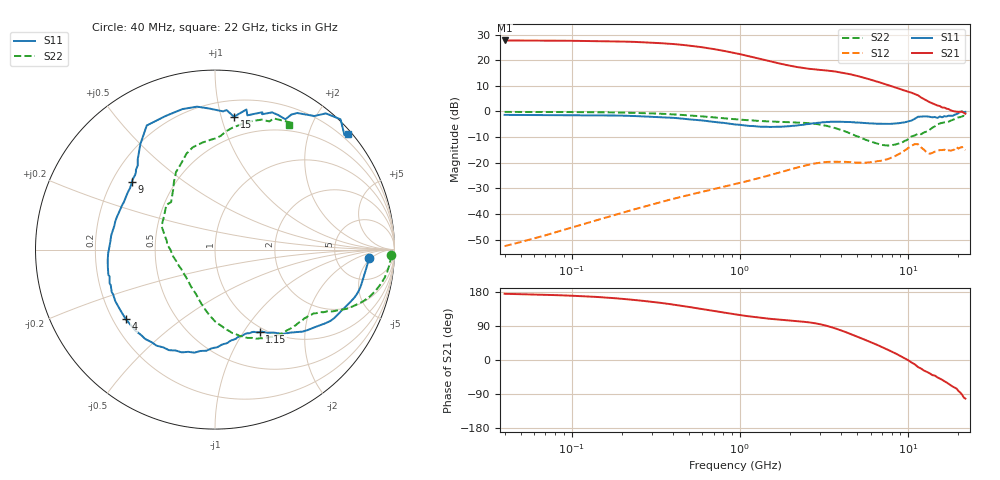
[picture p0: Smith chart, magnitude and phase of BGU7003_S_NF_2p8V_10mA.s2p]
!	Filename:	P:\Prog\Test\Noise\ATS_data\Testdata_Net\BGU7002	BGU7003	RN20082092\BGU7003_B1_high	freq_bias	loop_2.88V9.09mA_D.s2p
!	Date/Time:	Tue	16-Sep-08	9:24:41
!	BGU7003_B1_high	freq_bias	loop
!	bias	mode	1:00	Vout=	2.879	"V,"	Iout=	9.195	"mA,"	Vin=	3.955	"V,"	Iin=	0.8985	mA
!	Date/time	Mon	Aug	11	3:57:12	2008
!	Device	data	file	deembeded	for	feedlines	and	parallel
!	Original	file:	\BGU7002	BGU7003	RN20082092\BGU7003_B1_high	freq_bias	loop_2.88V9.09mA_R.s2p
!	Feed-files:	PR029V01_high	"frequency_140808_Feed1.s2p,"	PR029V01_high	frequency_140808_Feed2.s2p
!	Parallel-file:	PR029V01_high	frequency_140808_Par.s2p
#	MHz	S	MA	R	50
!	Freq-MHz	S11-mag	S11-arg	S21-mag	S21-arg	S12-mag	S12-arg	S22-mag	S22-arg
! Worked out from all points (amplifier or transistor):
!   160 points, 40 MHz to 22 GHz, reference 50 ohm
!   highest |S21| = 27.7 dB at 40 MHz (marker M1)
!   |S21| within 3 dB of that: start of sweep to 649.6 MHz
!   unconditionally stable (mu >= 1): nowhere
!   at 300 MHz: K = 0.29, MSG = 31.6 dB, |S12| = -36.3 dB
!   at 2.25 GHz: K = 0.58, MSG = 19.5 dB, |S12| = -21.7 dB
!   at 22 GHz: K = -0.08, MSG = 7.1 dB, |S12| = -15.1 dB
!   lowest NFmin = 0.58 dB at 400 MHz
!   S11 on the Smith chart (normalised r, x): 40 MHz: 12, -4; 1.15 GHz: 0.94, -1.18; 4 GHz: 0.25, -0.32; 9 GHz: 0.28, +0.33; 15 GHz: 0.33, +1.10; 22 GHz: 0.07, +2.66
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40  0.859 -3.3  24.36 174.8  0.00235 61.5  0.9811 -1.9
70  0.8522 -5.9  24.1 172.0  0.00383 71.2  0.9784 -3.6
120  0.8426 -10.4  23.83 168.1  0.00644 75.7  0.9713 -6.3
170  0.8364 -14.6  23.48 164.0  0.00901 76.2  0.9601 -8.9
220  0.8228 -18.7  23.02 159.8  0.01151 75.5  0.9457 -11.3
330  0.7766 -27.2  21.66 151.4  0.01662 73.1  0.9087 -16.0
450  0.7287 -34.9  20.06 143.0  0.02163 70.2  0.8586 -20.3
600  0.668 -43.2  17.93 134.2  0.02719 67.7  0.8027 -24.3
750  0.6107 -49.9  15.92 127.4  0.0322 65.8  0.7541 -26.9
950  0.5557 -56.4  13.67 120.2  0.03867 64.0  0.7064 -29.4
1150  0.5215 -61.5  11.86 115.0  0.04508 62.5  0.6735 -31.3
1350  0.5039 -66.0  10.47 111.1  0.05167 61.0  0.6514 -33.4
1650  0.5033 -72.3  8.969 107.1  0.06204 58.0  0.6316 -37.1
2150  0.5285 -84.9  7.456 102.8  0.07888 51.2  0.6112 -44.7
2700  0.5853 -101.3  6.729 98.1  0.09483 41.7  0.5832 -56.1
4000  0.6302 -142.2  5.781 78.3  0.1042 22.8  0.4359 -83.9
5400  0.6008 -174.4  4.628 55.7  0.1005 17.8  0.296 -106.9
7800  0.5725 152.4  3.205 24.8  0.1216 21.0  0.2174 -150.9
9000  0.5963 140.8  2.74 11.1  0.1519 18.9  0.2427 -175.2
11500  0.7892 118.8  2.067 -18.7  0.2301 -19.7  0.3683 137.5
15000  0.7477 81.9  1.309 -45.9  0.1696 -29.6  0.5575 106.6
22000  0.9832 41.1  0.9025 -102.0  0.1766 -81.5  0.8064 59.5
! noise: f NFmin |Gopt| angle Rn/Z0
400  0.585  0.235  10.52  0.122
1000  0.687  0.231  26.35  0.136
1500  0.773  0.23  39.55  0.142
1700  0.807  0.229  44.83  0.143
2200  0.893  0.23  58.03  0.144
3000  1.03  0.234  79.14  0.138
4400  1.27  0.251  116.1  0.117
5800  1.51  0.28  153.1  0.095
8000  1.888  0.351  -157.7  0.097
1.2e+04  2.574  0.557  -112.7  0.392
